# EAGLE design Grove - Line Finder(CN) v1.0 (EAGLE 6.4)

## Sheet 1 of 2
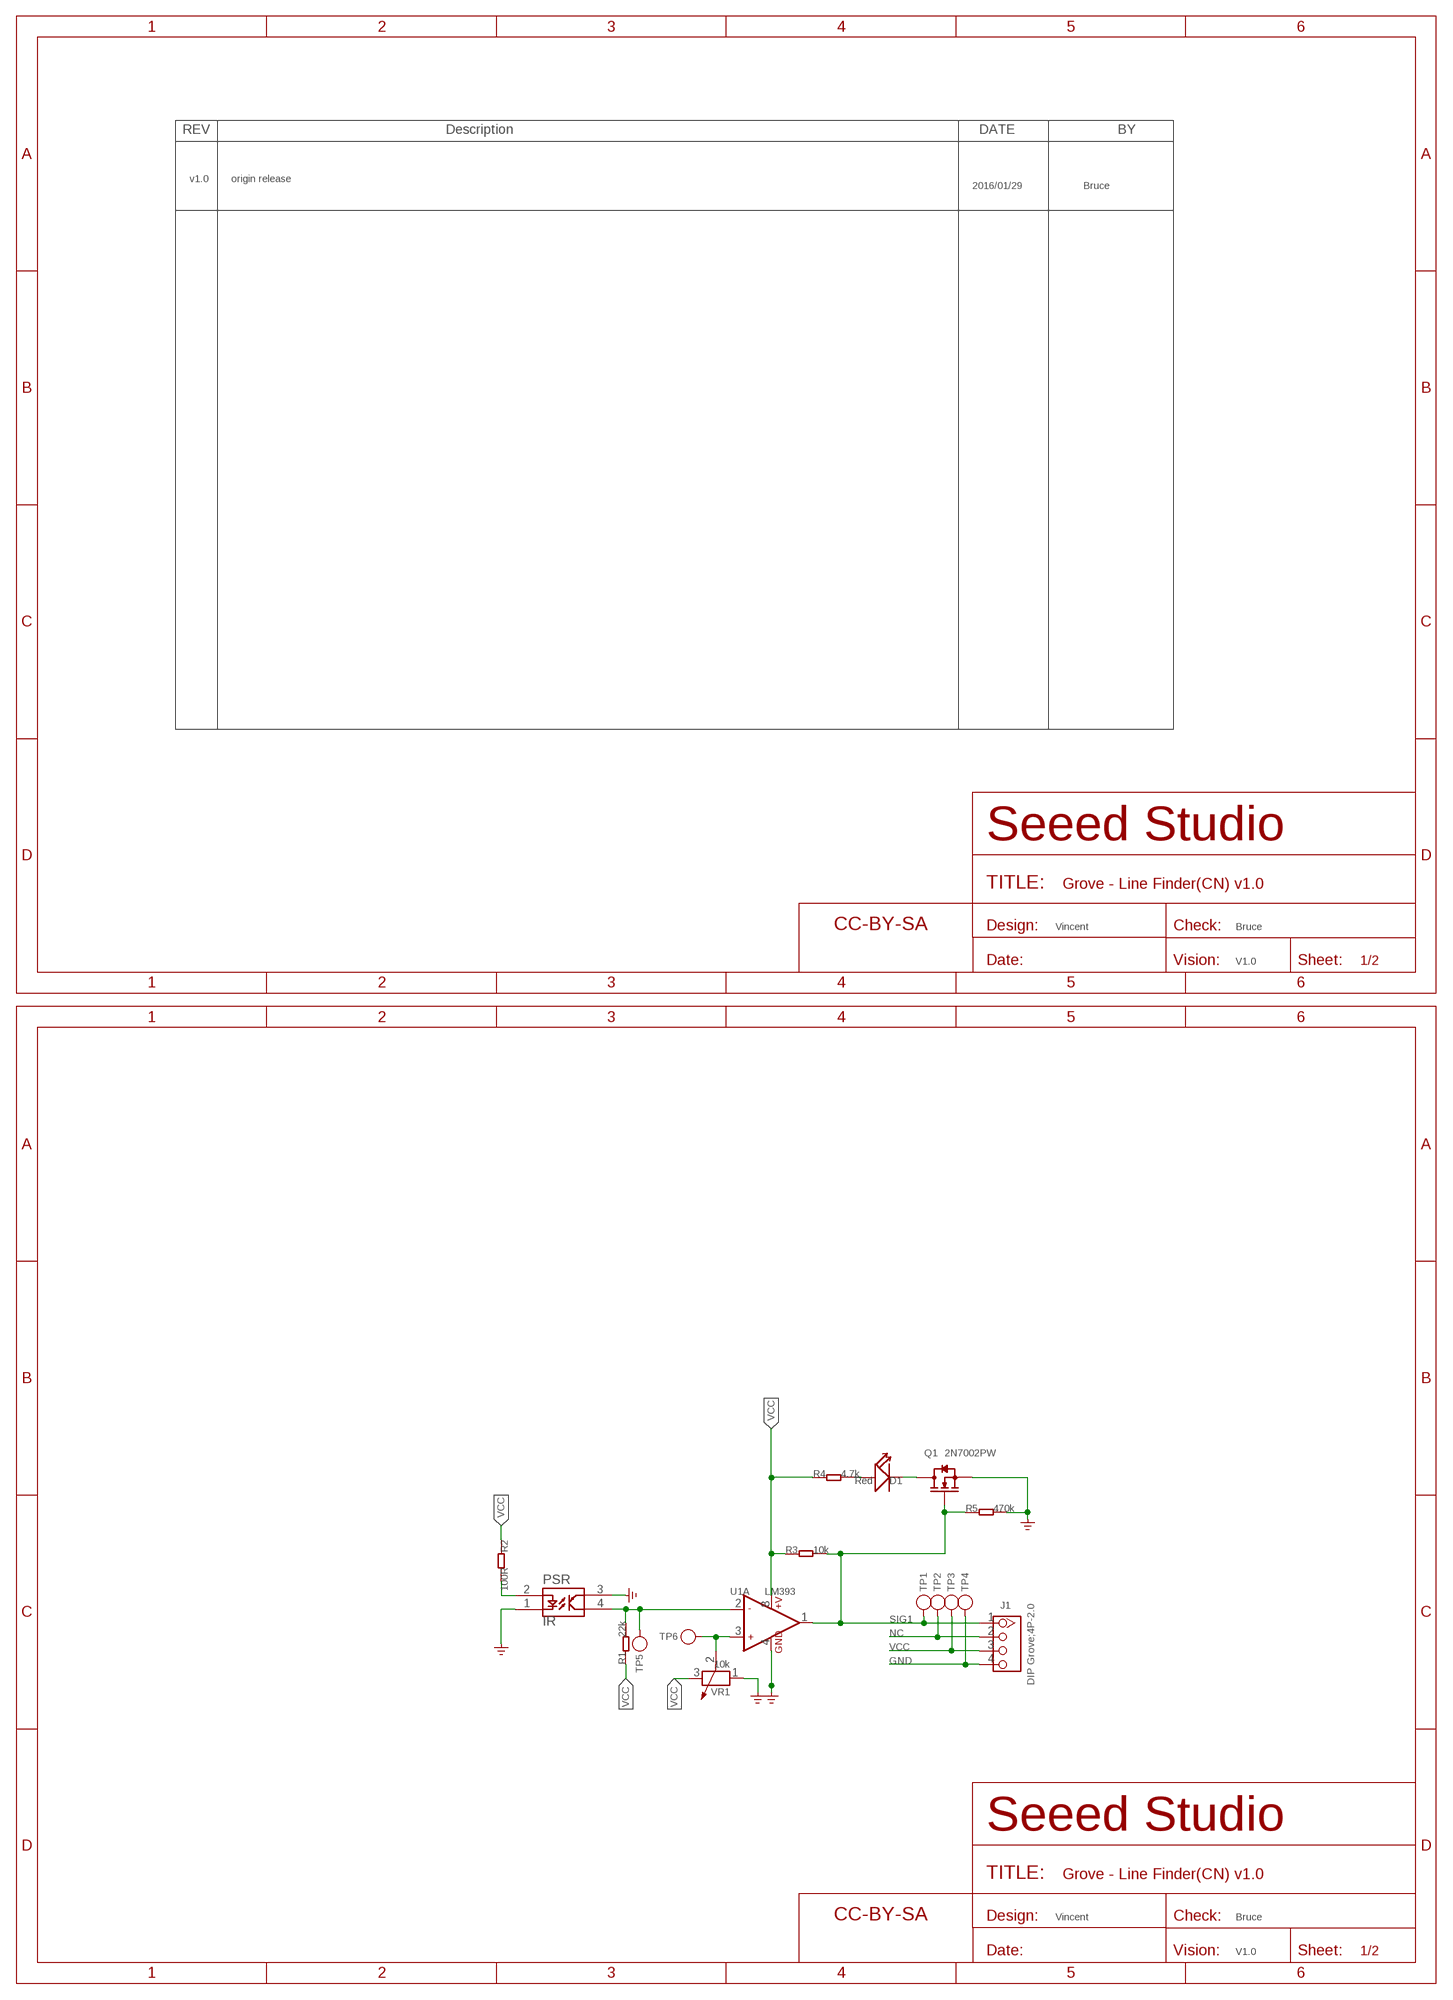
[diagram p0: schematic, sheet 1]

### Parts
D1  Red  LED'RIGHT'  [LED-SIDE-VIEW-0603-RIGHT]
FR1  SEEEDSTUDIO-OPEN-SCH-FRAME  [SEEEDSTUDIO-PCB-FRAME]
FR2  SEEEDSTUDIO-OPEN-SCH-FRAME  [SEEEDSTUDIO-PCB-FRAME]
J1  DIP Grove;4P-2.0  GROVE-CONNECTOR-DIP-2.0  [HW4-2.0]
PSR  PSR  [PSR]
Q1  2N7002PW  MOSFET-N'SOT23'  [SOT-23]
R1  22k  005-R0603_S  [0603_S]
R2  100R  005-R0603_S  [0603_S]
R3  10k  005-R0603_S  [0603_S]
R4  4.7k  005-R0603_S  [0603_S]
R5  470k  005-R0603_S  [0603_S]
TP1  TEST-POINT'4545'  [TP-D45MIL]
TP2  TEST-POINT'4545'  [TP-D45MIL]
TP3  TEST-POINT'4545'  [TP-D45MIL]
TP4  TEST-POINT'4545'  [TP-D45MIL]
TP5  TEST-POINT'4545'  [TP-D45MIL]
TP6  TEST-POINT'4545'  [TP-D45MIL]
U1  LM393  AMPLIFIER-LMV358'D'  [SOIC8-1.27-5X4MM]
VR1  10k  RES-ADJ'RTRIM3214W'  [ADJR3-SMD-4.6X3.7MM]

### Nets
GND: J1.4 PSR.1 PSR.3 Q1.2(S) R5.2 TP4.T U1.4(A:GND) VR1.1 ; supply symbol labelled GND_POWER
N$1: TP6.T U1.3(A:+IN1) VR1.2
N$2: PSR.4 R1.2 TP5.T U1.2(A:-IN1)
N$3: D1.1(+) R4.2
N$4: D1.2(-) Q1.3(D)
N$5: PSR.2 R2.2
NC: J1.2 TP2.T
SIG1: J1.1 Q1.1(G) R3.2 R5.1 TP1.T U1.1(A:OUT1)
VCC: J1.3 R1.1 R2.1 R3.1 R4.1 TP3.T U1.8(A:+V) VR1.3
Unconnected: U1.5(B:+IN2) U1.6(B:-IN2) U1.7(B:OUT2)

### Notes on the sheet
- v1.0 | origin release
- 2016/01/29 | Bruce
- Vincent | Bruce
- V1.0
- Vincent | Bruce
- V1.0

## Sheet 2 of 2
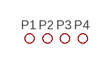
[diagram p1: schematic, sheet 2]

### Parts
P1  PAD-MARK'ANNULAR'  [ROUND-MARK-1.0]
P2  PAD-MARK'ANNULAR'  [ROUND-MARK-1.0]
P3  PAD-MARK'ANNULAR'  [ROUND-MARK-1.0]
P4  PAD-MARK'ANNULAR'  [ROUND-MARK-1.0]

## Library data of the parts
D1 = Discrete-new:LED
FR1 FR2 = moudle-new:SEEEDSTUDIO-OPEN-SCH-FRAME
J1 = Connector-new:GROVE-CONNECTOR-DIP: 4P-2.0:320110033;4P-2.0-90D:320110034
P1-P4 = Discrete-new:PAD-MARK; PARTNO: DNP
PSR = IR:PSR*
Q1 = Discrete-new:MOSFET-N
R1-R5 = Discrete:005-R*
TP1-TP6 = Discrete-new:TEST-POINT; PARTNO: DNP
U1 = IC-new:AMPLIFIER-LMV358: SOIC-8:310020002;MSOP-8:310020007
VR1 = Discrete-new:RES-ADJ: Potentiometer

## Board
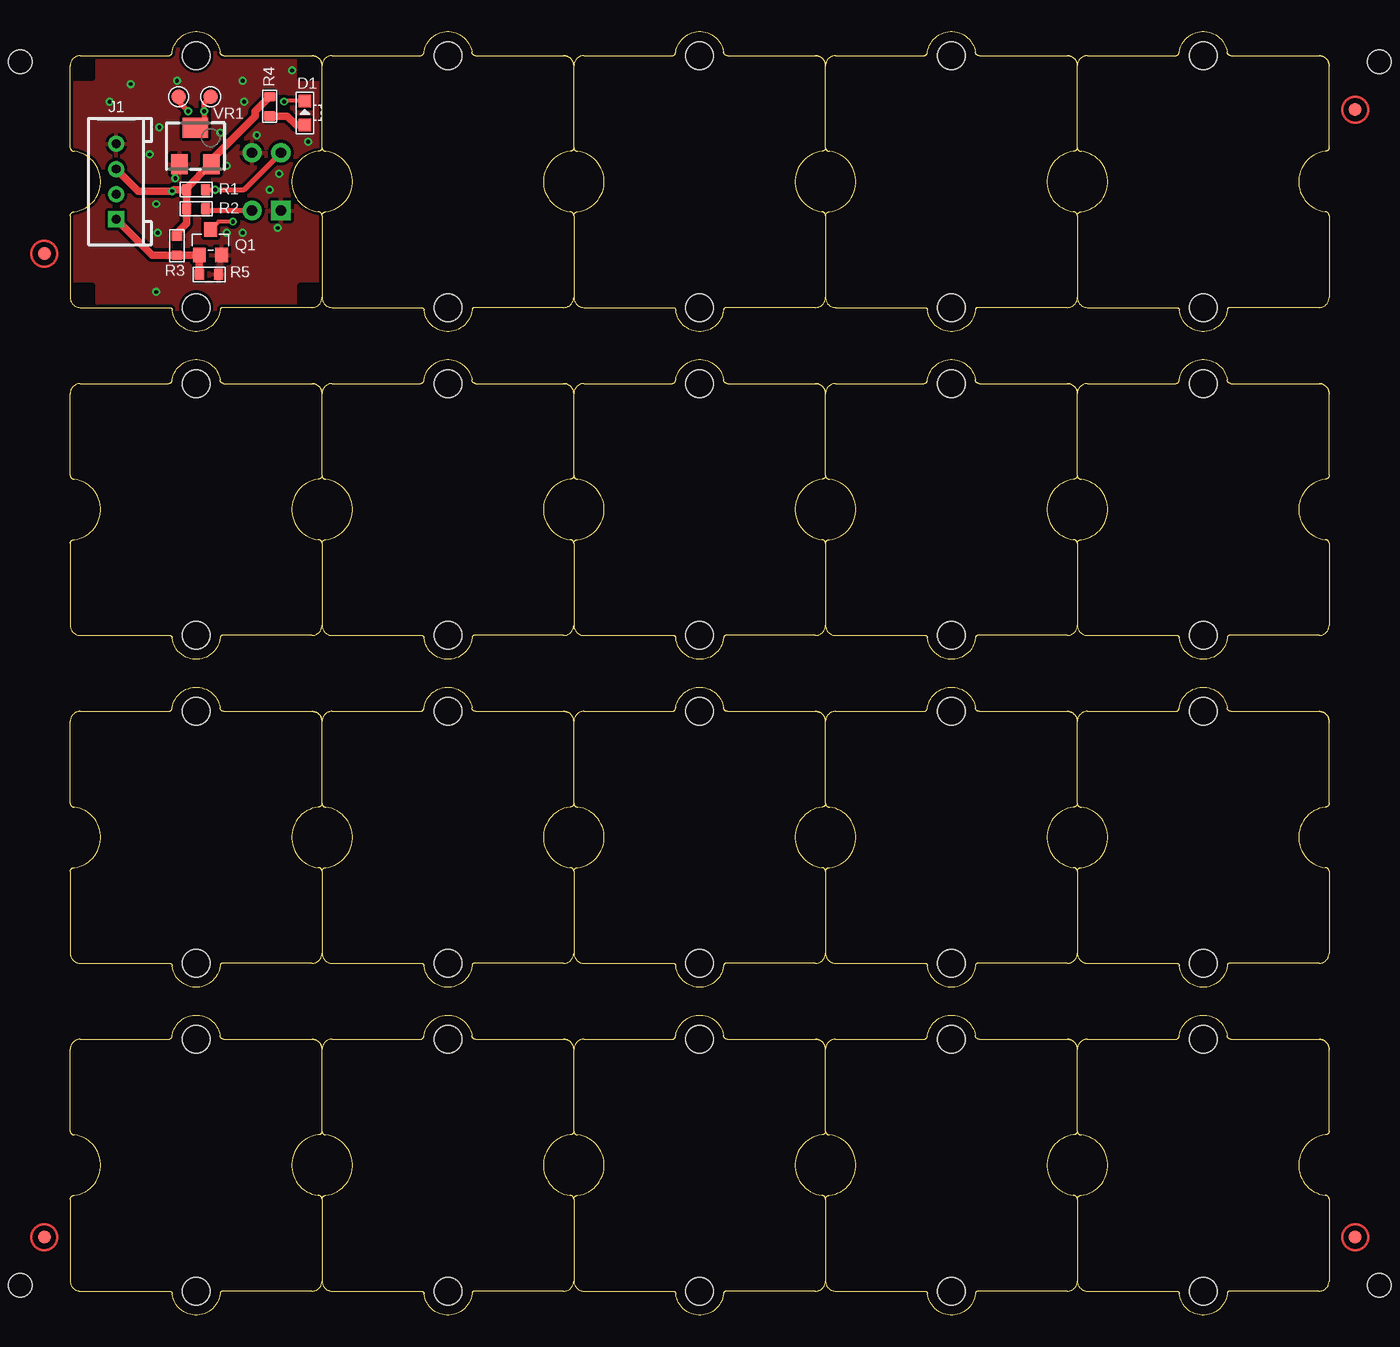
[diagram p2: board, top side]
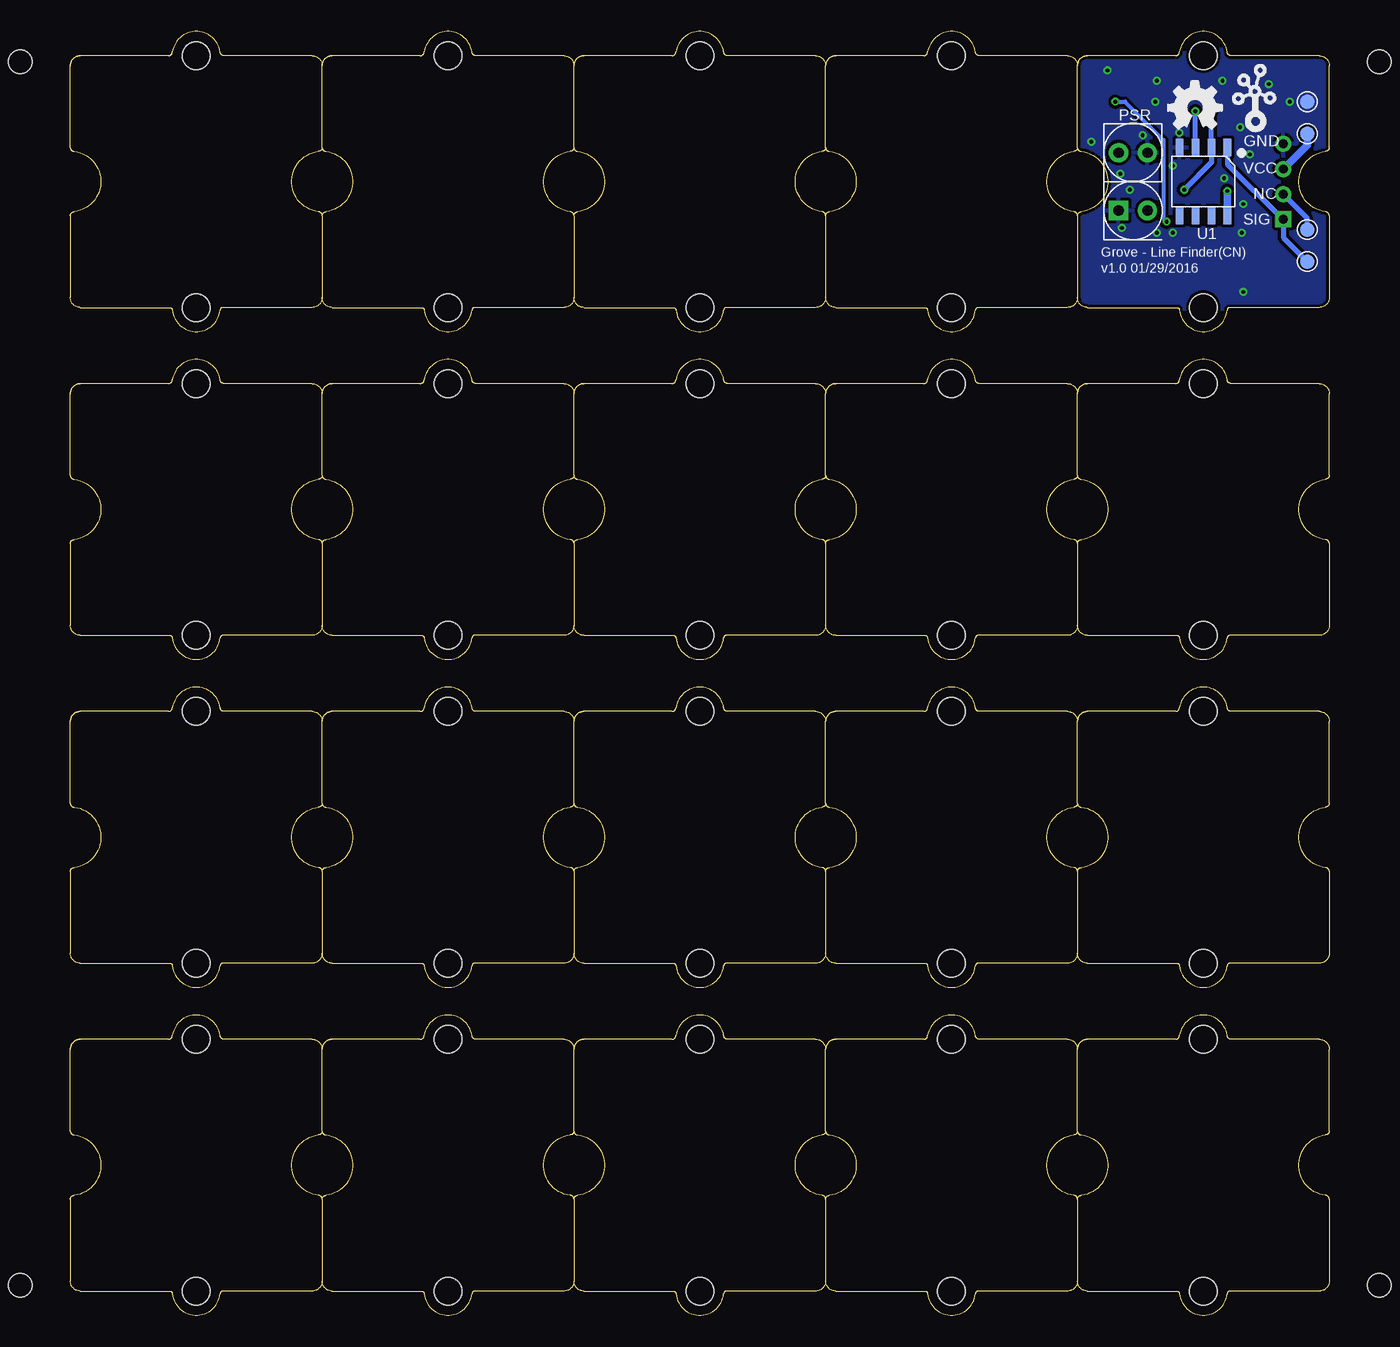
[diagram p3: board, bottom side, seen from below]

Size 100 x 101.93 mm. Coordinates in mm from the lower left corner, seen from the top.
Copper layers (1*16): Top 0.035mm / dielectric 1.5mm / Bottom 0.035mm
Design rules "SeeedStudio_2layer_DRU_no_angle_20140221": minimum track width 6mil, minimum drill 12mil, track to track 6mil, track to pad 6mil, pad to pad 6mil, via to via 6mil, smd to smd 0mil, copper to edge 10mil, drill to drill 10mil, minimum pad ring 10mil, minimum via ring 6mil, stop-mask expansion 2mil, vias tented up to drill 25mil, thermal gap 10mil
Holes 1.91 mm at -3.97,2.38 -3.97,99.54 103.98,99.54 103.98,2.38
tRestrict: area 28.2,124.9 to 29.3,126.2
bRestrict: area 28.2,124.9 to 29.3,126.2

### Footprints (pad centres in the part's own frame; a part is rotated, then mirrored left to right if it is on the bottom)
LED-SIDE-VIEW-0603-RIGHT = smd 1 x 1: 1 0,-0.95; 2 0,0.95
HW4-2.0 = drill 0.7 pad 1.27 square: 1 -3,0 | drill 0.7 pad 1.27: 2 -1,0; 3 1,0; 4 3,0
ROUND-MARK-1.0 = smd 1.016 x 1.016: P$1 0,0
PSR = drill 0.813 pad 1.524 square: 1 -2.3,1.15 | drill 0.813 pad 1.524: 2 -2.3,-1.15; 3 2.3,-1.15; 4 2.3,1.15
SOT-23 = smd 1.016 x 1.143: 1 -0.889,-1.016; 2 0.889,-1.016; 3 0,1.016
0603_S = smd 0.762 x 0.889: 1 -0.762,0; 2 0.762,0
TP-D45MIL = smd 1.143 x 1.143: T 0,0
SOIC8-1.27-5X4MM = smd 0.6 x 1.4: 1 -1.905,-2.7; 2 -0.635,-2.7; 3 0.635,-2.7; 4 1.905,-2.7; 5 1.905,2.7; 6 0.635,2.7; 7 -0.635,2.7; 8 -1.905,2.7
GROVE-1*1-TEST-PLATFORM = hole 2.2: 0,-10; 0,10
ADJR3-SMD-4.6X3.7MM = smd 1.3 x 1.6: 1 -1.275,-1.45; 3 1.275,-1.45 | smd 2 x 1.6: 2 0,1.45

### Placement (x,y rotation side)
D1  18.64,95.47 0 top
FR1  not placed on the board
FR2  not placed on the board
J1  3.65,90.01 90 top
P1  -2.06,6.19 0 top
P2  102.08,6.19 0 top
P3  -2.06,84.3 0 top
P4  102.08,95.73 0 top
PSR  15.59,90.01 90 bottom
Q1  11.14,85.19 0 top
R1  10,89.38 0 top
R2  10,87.85 0 top
R3  8.48,84.93 270 top
R4  15.84,95.98 270 top
R5  11.02,82.65 0 top
TP1  1.74,83.66 0 bottom
TP2  1.74,86.2 0 bottom
TP3  1.74,93.82 0 bottom
TP4  1.74,96.36 0 bottom
TP5  8.6,96.74 270 top
TP6  11.14,96.74 270 top
U1  10,90.01 180 bottom
U$5  [GROVE-1*1-TEST-PLATFORM]  10,90.01 0 top
U$9  [GROVE-1*1-TEST-PLATFORM]  30,90.01 0 top
U$10  [GROVE-1*1-TEST-PLATFORM]  50,90.01 0 top
U$11  [GROVE-1*1-TEST-PLATFORM]  70,90.01 0 top
U$12  [GROVE-1*1-TEST-PLATFORM]  90,90.01 0 top
U$13  [GROVE-1*1-TEST-PLATFORM]  30,63.98 0 top
U$14  [GROVE-1*1-TEST-PLATFORM]  50,63.98 0 top
U$15  [GROVE-1*1-TEST-PLATFORM]  70,63.98 0 top
U$16  [GROVE-1*1-TEST-PLATFORM]  90,63.98 0 top
U$17  [GROVE-1*1-TEST-PLATFORM]  10,63.98 0 top
U$18  [GROVE-1*1-TEST-PLATFORM]  30,37.94 0 top
U$19  [GROVE-1*1-TEST-PLATFORM]  50,37.94 0 top
U$20  [GROVE-1*1-TEST-PLATFORM]  70,37.94 0 top
U$21  [GROVE-1*1-TEST-PLATFORM]  90,37.94 0 top
U$22  [GROVE-1*1-TEST-PLATFORM]  10,37.94 0 top
U$23  [GROVE-1*1-TEST-PLATFORM]  30,11.91 0 top
U$24  [GROVE-1*1-TEST-PLATFORM]  50,11.91 0 top
U$25  [GROVE-1*1-TEST-PLATFORM]  70,11.91 0 top
U$26  [GROVE-1*1-TEST-PLATFORM]  90,11.91 0 top
U$27  TWIGLOGOTWIGLOGO_SMALL  [TWIGLOGO_SMALL]  8.1,93.82 0 bottom
U$28  [GROVE-1*1-TEST-PLATFORM]  10,11.91 0 top
U$29  [OSHW_FILLX150_NOTEXT]  12.79,94.2 0 bottom
VR1  9.95,92.83 0 top

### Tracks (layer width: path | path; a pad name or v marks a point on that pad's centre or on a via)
GND  (via drill 0.3 pad 0.64)
  other vias: 3.14,96.36 16.48,86.33 6.83,88.24 8.35,90.27 11.9,93.89 17.62,98.84 13.68,85.95 12.41,85.95 6.83,81.25 6.95,85.95 6.32,92.17 7.08,94.33 4.79,97.76 8.48,98.01 13.68,98.01 13.81,96.36 12.41,91.28 14.83,93.7 15.84,89.38 16.6,90.65 18.89,93.19
  pour Top (isolate 0.254): -0.92,100.68 20.67,100.68 20.67,79.6 -0.92,79.6
  pour Bottom (isolate 0.254): -0.92,100.68 20.67,100.68 20.67,79.6 -0.92,79.6
N$1  (via drill 0.3 pad 0.64)
  Top 0.406: TP6.T 10.63,96.24 v10.63,95.6 10.63,94.84 10.13,94.33 10,94.33 VR1.2
  Bottom 0.406: U1.3 v10.63,95.6
N$2  (via drill 0.3 pad 0.64)
  Top 0.406: PSR.4 13.8,89.38 v11.52,89.38 R1.2 | TP5.T 8.6,96.36 v9.37,95.6
  Bottom 0.406: v9.37,95.6 U1.2 9.37,91.54 v11.52,89.38
N$3
  Top 0.61: D1.1 17.93,94.52 17.24,95.22 R4.2
N$4  (via drill 0.3)
  Top 0.305: D1.2 17.05,96.42 v16.98,96.36 | v12.92,86.84 11.78,86.84 Q1.3
  Bottom 0.305: v16.98,96.36 16.22,96.36 13.18,93.32 13.18,87.09 v12.92,86.84
N$5
  Top 0.406: PSR.2 10.9,87.71 R2.2
NC
  Bottom 0.406: TP2.T 1.74,87.11 J1.2
SIG1
  Top 0.61: R5.1 Q1.1 R3.2 6.49,84.17 J1.1
  Bottom 0.406: TP1.T 3.65,85.57 J1.1 3.7,87.01 8.1,91.41 U1.1
VCC  (via drill 0.3 pad 0.64)
  Top 0.61: R2.1 9.24,87.6 | R2.1 R1.1 | R1.1 9.24,89.51 11.12,91.38 VR1.3 11.22,91.75 14.7,95.22 14.7,95.6 R4.1 | R1.1 8.21,89.38 v8.1,89.27 5.4,89.27 J1.3 | R3.1 8.48,85.95 9.24,86.71 R2.1
  Bottom 0.61: U1.8 v8.1,89.27 | TP3.T 1.74,92.92 J1.3

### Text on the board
bPlace: GND | VCC | NC | SIG | Grove - Line Finder(CN) | v1.0 01/29/2016

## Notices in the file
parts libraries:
moudle-new: This work is licensed under the Creative Commons Attribution 4.0 International License.
To view a copy of this license,visit:
http://creativecommons.org/licenses/by-sa/4.0
moudle-new: CC-BY-SA
